(* Logix 5000 AddOnInstructionDefinition export Banner_K50Pro_Compact_Aud_Param_v4; software revision 33.03 *)

TYPE Banner_IOL_Port_v4 :   // UDT that has all of the data items necessary to communicate with a specific Port on a IO-Link Master
STRUCT
   Port_Controlled : INT;   // Each bit represents a port on an IO-Link Master. Set to 1 to tell AOI to control that port.
   Port_Activate : INT;   // Each bit represents a port on an IO-Link Master. When ON that port will process any commands in queue.
   Port_Read : INT;   // Each bit represents a port on an IO-Link Master. Used to determine when device AOI has requested a Read command.
   Port_Write : INT;   // Each bit represents a port on an IO-Link Master. Used to determine when device AOI has requested a Write command.
   Port_RW_Complete : INT;   // Each bit represents a port on an IO-Link Master. Tells device AOI that Read or Write request has been completed.
   Port_Device_Read : INT;
   Data_Transfer : SINT[190];   // Array to transfer data from IO-Master to device AOIs.
END_STRUCT
END_TYPE

TYPE Banner_K50ComAud_Audible_Tone_v4 :   // UDT for K50 Compact Audible with the Custom Audible Tone structure.
STRUCT
   Audible_Type : SINT;   // 0 = Beep, 1 = Sweep, 2 = Tone.
   Sweep_Type : SINT;   // 0 = Up, 1 = Down, 2 = Up Down, 3 = Down Up.
   Frequency1 : SINT;   // 0 = Off, 1 = Low, 2 = Standard, 3 =High.
   Frequency2 : SINT;   // 0 = Off, 1 = Low, 2 = Standard, 3 =High.
END_STRUCT
END_TYPE

TYPE Banner_K50ComAud_Direct_v4 :   // UDT with all of the Direct Parameters for K50 Compact Audible.
STRUCT
   Master_Cycle_Time : INT;
   Min_Cycle_Time : INT;
   M_Sequence_Capability : INT;
   IO_Link_Version_ID : INT;
   Process_Data_Input_Length : INT;
   Process_Data_Output_Length : INT;
   Combined_Vendor_ID : DINT;   // IO-Link Vendor ID
   Vendor_ID1 : INT;
   Vendor_ID2 : INT;
   Combined_Device_ID : DINT;   // IO-Link Device ID
   Device_ID1 : INT;
   Device_ID2 : INT;
   Device_ID3 : INT;
END_STRUCT
END_TYPE

TYPE Banner_K50ComAud_RD_v4 :   // UDT with all of the Read only parameters for K50 Compact Audible.
STRUCT
   Direct : Banner_K50ComAud_Direct_v4;
   Serial_Number : STRING;
END_STRUCT
END_TYPE

TYPE Banner_K50ComAud_SP_v4 :   // UDT for K50 Compact Audible with the State Parameters structure.
STRUCT
   Audible_Feedback : SINT;   // 0 = Off, 3 = On.
   Audible_Volume : SINT;   // 0 = Off, 1 = Low, 2 = Medium, 3 = High.
   Audible_Type : SINT;   // 0 = Pulse, 1 = Wobble, 2 = Strobe, 3 = Whoop, 4 = Stcatto, 5 = Siren, 6 = Continuous 1, 7 = Continuous 2, 9 = Jingle, 10 = Melody 1, 11 = Melody 2, 12 = Melody 3, 13 = Custom.
END_STRUCT
END_TYPE

TYPE Banner_K50ComAud_v4 :   // UDT with all of the parameters for K50 Compact Audible.
STRUCT
   Initial_Global_Read : BOOL;   // Determines if all of the IO-Link data has been read into the PLC yet
   Command : INT;   // Value placed in here will activate a read or write to a specifc IO-Link Index
   Read : Banner_K50ComAud_RD_v4;   // All read data
   Write : Banner_K50ComAud_WD_v4;   // All data that can be written to.
   Reset : BOOL;
END_STRUCT
END_TYPE

TYPE Banner_K50ComAud_WD_v4 :   // UDT that stores the Write Data for a K50 Compact Audible.
STRUCT
   System_Command : INT;   // See IODD file for list of commands that can be activated via the System Command interface
   Parameter_Access_Lock : SINT;   // Write access to all read/write parameters is block when this bit is ON.
   Data_Storage_Lock : SINT;   // Data storage mechanism is inhibited when bit is ON.
   Local_Parameterization_Lock : SINT;   // Parameteriation via local control elementes is inhibited.
   Local_User_Interface_Lock : SINT;   // Operation of the hmi on the device is disabled.
   Operation_Mode : SINT;   // 0 = Multicolor, 1 = Four State Full Logic, 2 = Advanced, 3 = LED Control, 4 = Demo.
   State_Parameters : Banner_K50ComAud_SP_v4[5];   // State Parameters. 1 through 4 will have values.
   Aud_Tone : Banner_K50ComAud_Audible_Tone_v4;   // 0-255. Custom 1 Red.
END_STRUCT
END_TYPE

ADD_ON_INSTRUCTION Banner_K50Pro_Compact_Aud_Param_v4   (* revision 4.0, vendor Banner Engineering *)
// AOI to read and write parameter data to an IO-Link K50 Pro Compact Audible.
VAR_IN_OUT
   K50 : Banner_K50ComAud_v4; {required}
   Port_Data : Banner_IOL_Port_v4; {required}
END_VAR
VAR_INPUT
   Port : DINT; {required}
END_VAR
VAR
   Local_Control : DINT; {access None}
   Global_Read_Command_Value : INT; {access None}
   Global_Write_Command_Value : INT; {access None}
   Command_Being_Processed : BOOL; {access None}
   Index_Write_Control : DINT; {access None}
   Index_Write_Inprocess : INT; {access None}
   Temp_Excess_Gain : DINT[2]; {access None}
   Inprocess_Index : DINT; {access None}
   SP_Index : DINT; {access None}   // State Parameters Index
   SP_Write_Index : DINT; {access None}
   SP_R_Index : DINT; {access None}
   SP_W_Index : DINT; {access None}
END_VAR

ROUTINE Logic   (* ladder *)
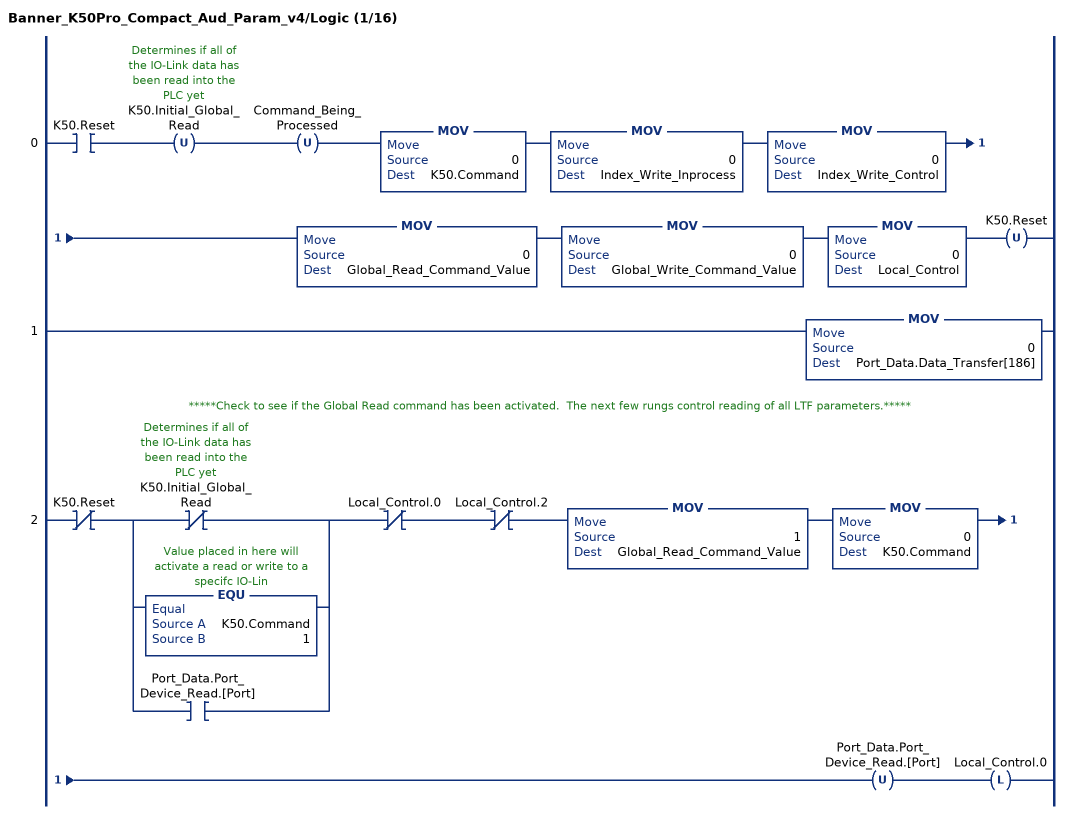
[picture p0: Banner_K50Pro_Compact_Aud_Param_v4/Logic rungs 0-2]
   0: XIC(K50.Reset)OTU(K50.Initial_Global_Read)OTU(Command_Being_Processed)MOV(0,K50.Command)MOV(0,Index_Write_Inprocess)MOV(0,Index_Write_Control)MOV(0,Global_Read_Command_Value)MOV(0,Global_Write_Command_Value)MOV(0,Local_Control)OTU(K50.Reset);
   1: MOV(0,Port_Data.Data_Transfer[186]);
   // *****Check to see if the Global Read command has been activated.  The next few rungs control reading of all LTF parameters.*****
   2: XIO(K50.Reset)[XIO(K50.Initial_Global_Read) ,EQU(K50.Command,1) ,XIC(Port_Data.Port_Device_Read.[Port]) ]XIO(Local_Control.0)XIO(Local_Control.2)MOV(1,Global_Read_Command_Value)MOV(0,K50.Command)OTU(Port_Data.Port_Device_Read.[Port])OTL(Local_Control.0);
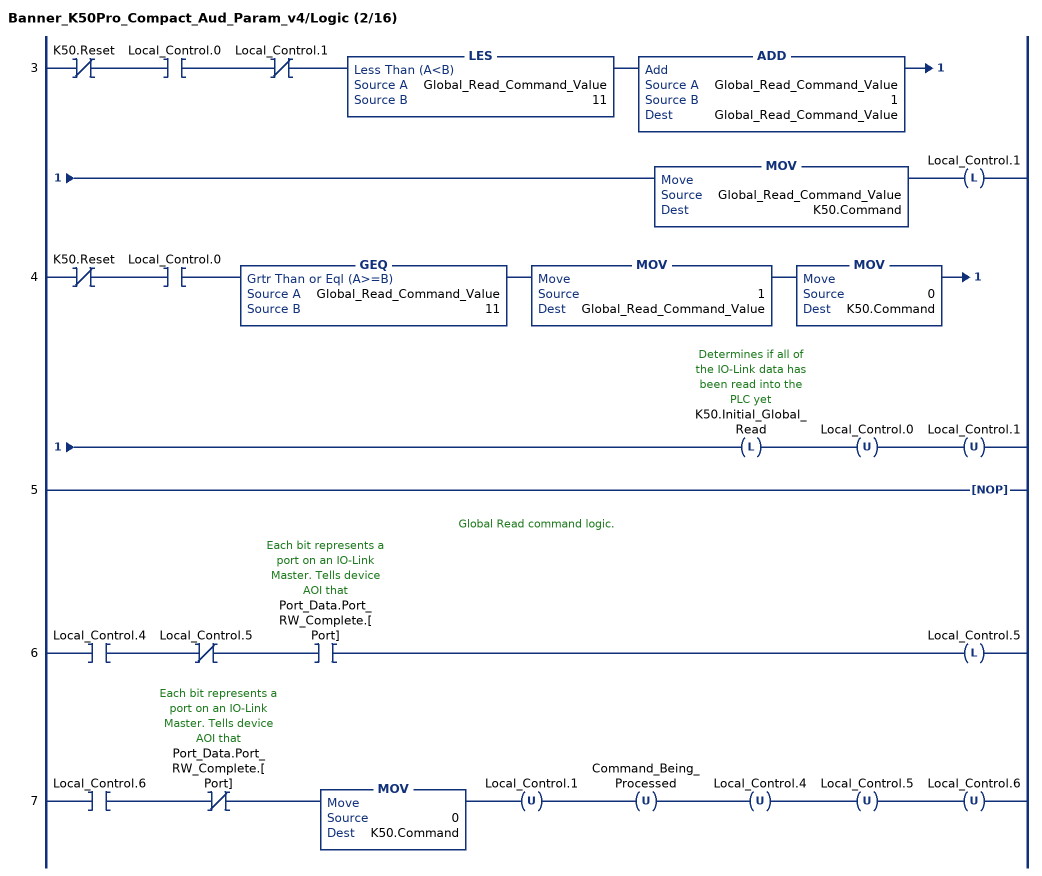
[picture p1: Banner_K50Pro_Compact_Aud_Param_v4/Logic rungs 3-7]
   3: XIO(K50.Reset)XIC(Local_Control.0)XIO(Local_Control.1)LES(Global_Read_Command_Value,11)ADD(Global_Read_Command_Value,1,Global_Read_Command_Value)MOV(Global_Read_Command_Value,K50.Command)OTL(Local_Control.1);
   4: XIO(K50.Reset)XIC(Local_Control.0)GEQ(Global_Read_Command_Value,11)MOV(1,Global_Read_Command_Value)MOV(0,K50.Command)OTL(K50.Initial_Global_Read)OTU(Local_Control.0)OTU(Local_Control.1);
   5: NOP();
   // Global Read command logic.
   6: XIC(Local_Control.4)XIO(Local_Control.5)XIC(Port_Data.Port_RW_Complete.[Port])OTL(Local_Control.5);
   7: XIC(Local_Control.6)XIO(Port_Data.Port_RW_Complete.[Port])MOV(0,K50.Command)OTU(Local_Control.1)OTU(Command_Being_Processed)OTU(Local_Control.4)OTU(Local_Control.5)OTU(Local_Control.6);
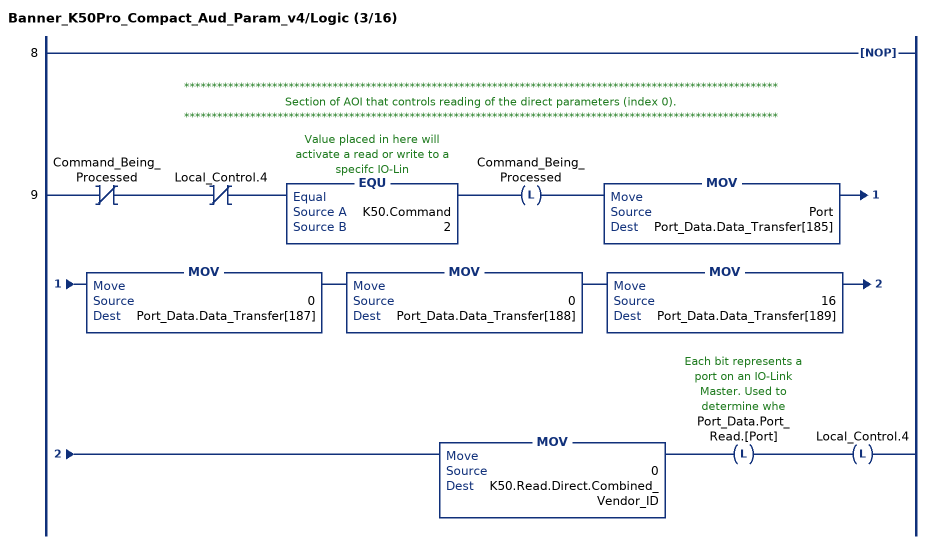
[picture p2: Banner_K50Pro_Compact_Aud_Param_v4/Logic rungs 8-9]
   8: NOP();
   // ************************************************************************************************************
   // Section of AOI that controls reading of the direct parameters (index 0).
   // ************************************************************************************************************
   9: XIO(Command_Being_Processed)XIO(Local_Control.4)EQU(K50.Command,2)OTL(Command_Being_Processed)MOV(Port,Port_Data.Data_Transfer[185])MOV(0,Port_Data.Data_Transfer[187])MOV(0,Port_Data.Data_Transfer[188])MOV(16,Port_Data.Data_Transfer[189])MOV(0,K50.Read.Direct.Combined_Vendor_ID)OTL(Port_Data.Port_Read.[Port])OTL(Local_Control.4);
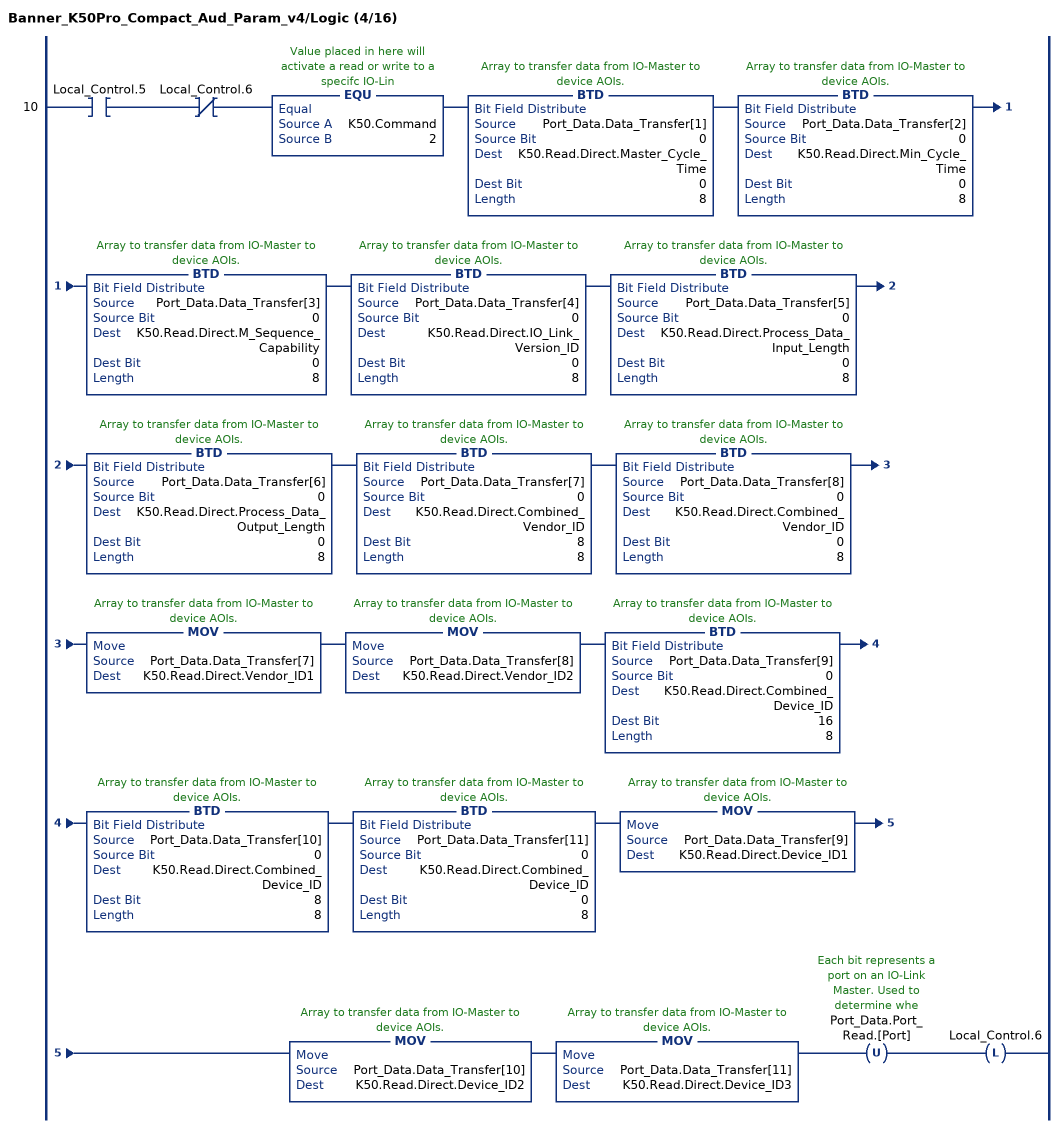
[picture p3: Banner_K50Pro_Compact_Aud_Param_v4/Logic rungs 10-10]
   10: XIC(Local_Control.5)XIO(Local_Control.6)EQU(K50.Command,2)BTD(Port_Data.Data_Transfer[1],0,K50.Read.Direct.Master_Cycle_Time,0,8)BTD(Port_Data.Data_Transfer[2],0,K50.Read.Direct.Min_Cycle_Time,0,8)BTD(Port_Data.Data_Transfer[3],0,K50.Read.Direct.M_Sequence_Capability,0,8)BTD(Port_Data.Data_Transfer[4],0,K50.Read.Direct.IO_Link_Version_ID,0,8)BTD(Port_Data.Data_Transfer[5],0,K50.Read.Direct.Process_Data_Input_Length,0,8)BTD(Port_Data.Data_Transfer[6],0,K50.Read.Direct.Process_Data_Output_Length,0,8)BTD(Port_Data.Data_Transfer[7],0,K50.Read.Direct.Combined_Vendor_ID,8,8)BTD(Port_Data.Data_Transfer[8],0,K50.Read.Direct.Combined_Vendor_ID,0,8)MOV(Port_Data.Data_Transfer[7],K50.Read.Direct.Vendor_ID1)MOV(Port_Data.Data_Transfer[8],K50.Read.Direct.Vendor_ID2)BTD(Port_Data.Data_Transfer[9],0,K50.Read.Direct.Combined_Device_ID,16,8)BTD(Port_Data.Data_Transfer[10],0,K50.Read.Direct.Combined_Device_ID,8,8)BTD(Port_Data.Data_Transfer[11],0,K50.Read.Direct.Combined_Device_ID,0,8)MOV(Port_Data.Data_Transfer[9],K50.Read.Direct.Device_ID1)MOV(Port_Data.Data_Transfer[10],K50.Read.Direct.Device_ID2)MOV(Port_Data.Data_Transfer[11],K50.Read.Direct.Device_ID3)OTU(Port_Data.Port_Read.[Port])OTL(Local_Control.6);
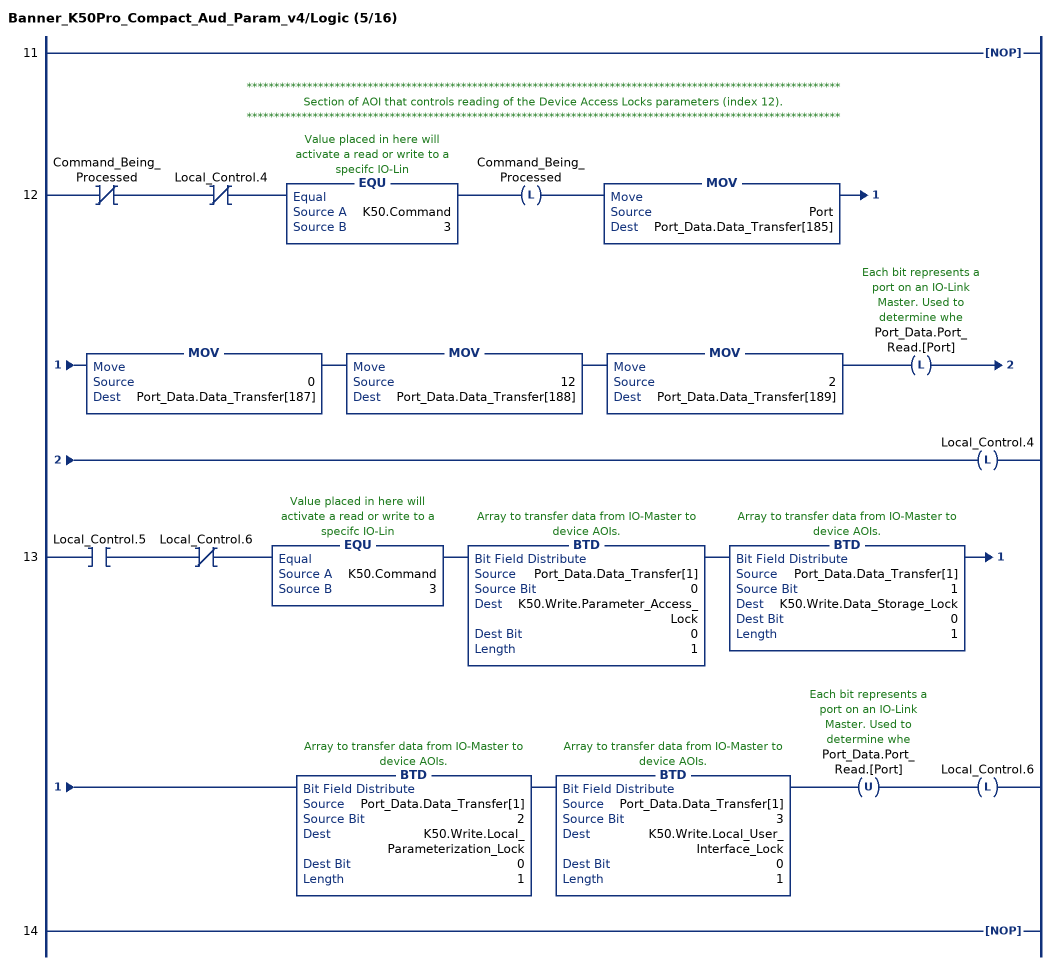
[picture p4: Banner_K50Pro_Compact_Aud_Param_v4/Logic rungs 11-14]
   11: NOP();
   // ************************************************************************************************************
   // Section of AOI that controls reading of the Device Access Locks parameters (index 12).
   // ************************************************************************************************************
   12: XIO(Command_Being_Processed)XIO(Local_Control.4)EQU(K50.Command,3)OTL(Command_Being_Processed)MOV(Port,Port_Data.Data_Transfer[185])MOV(0,Port_Data.Data_Transfer[187])MOV(12,Port_Data.Data_Transfer[188])MOV(2,Port_Data.Data_Transfer[189])OTL(Port_Data.Port_Read.[Port])OTL(Local_Control.4);
   13: XIC(Local_Control.5)XIO(Local_Control.6)EQU(K50.Command,3)BTD(Port_Data.Data_Transfer[1],0,K50.Write.Parameter_Access_Lock,0,1)BTD(Port_Data.Data_Transfer[1],1,K50.Write.Data_Storage_Lock,0,1)BTD(Port_Data.Data_Transfer[1],2,K50.Write.Local_Parameterization_Lock,0,1)BTD(Port_Data.Data_Transfer[1],3,K50.Write.Local_User_Interface_Lock,0,1)OTU(Port_Data.Port_Read.[Port])OTL(Local_Control.6);
   14: NOP();
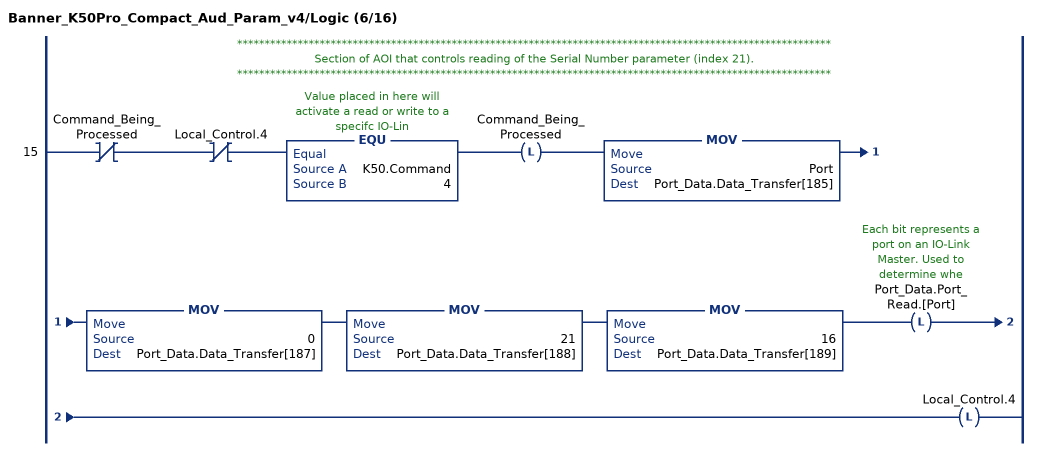
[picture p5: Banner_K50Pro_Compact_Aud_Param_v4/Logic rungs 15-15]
   // ************************************************************************************************************
   // Section of AOI that controls reading of the Serial Number parameter (index 21).
   // ************************************************************************************************************
   15: XIO(Command_Being_Processed)XIO(Local_Control.4)EQU(K50.Command,4)OTL(Command_Being_Processed)MOV(Port,Port_Data.Data_Transfer[185])MOV(0,Port_Data.Data_Transfer[187])MOV(21,Port_Data.Data_Transfer[188])MOV(16,Port_Data.Data_Transfer[189])OTL(Port_Data.Port_Read.[Port])OTL(Local_Control.4);
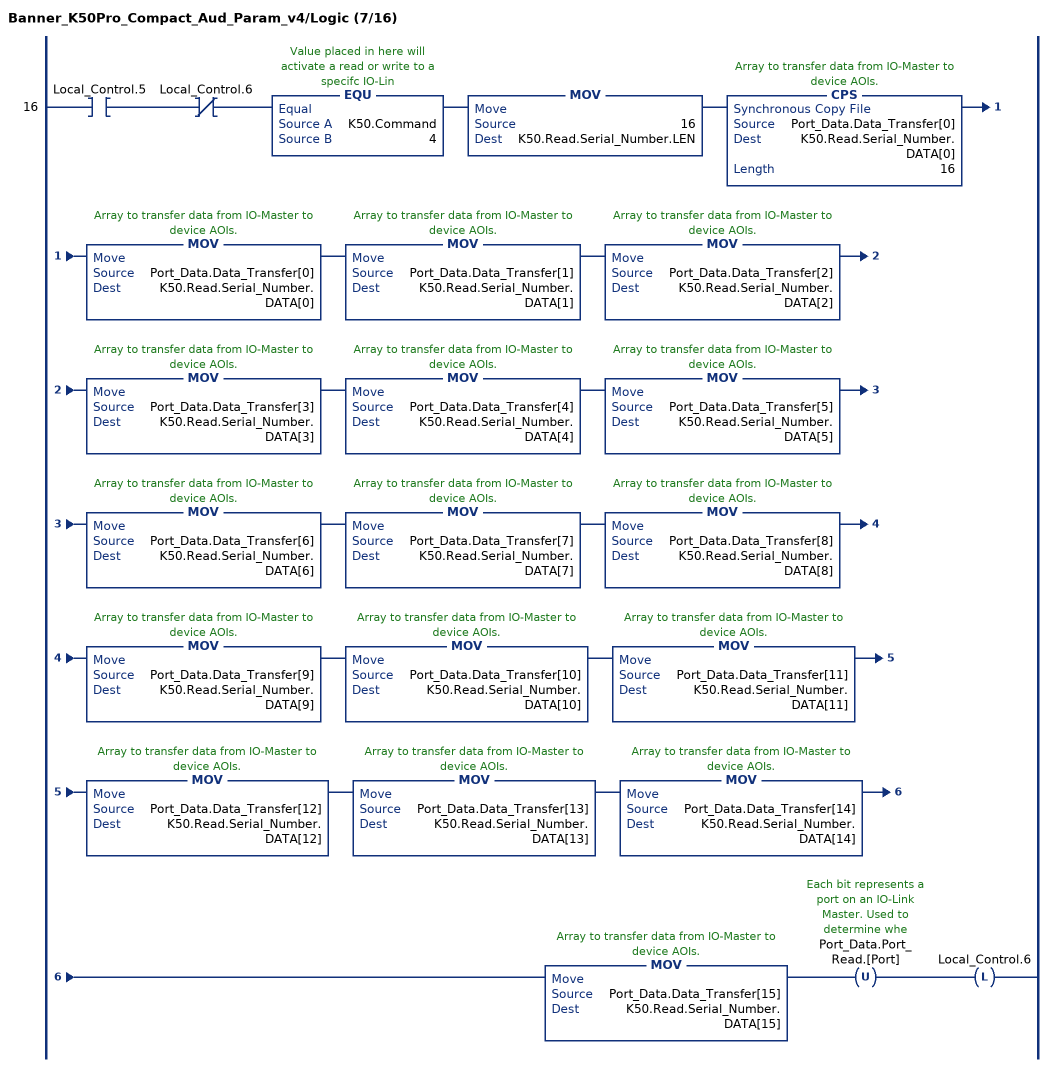
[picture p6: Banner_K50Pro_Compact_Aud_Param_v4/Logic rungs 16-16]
   16: XIC(Local_Control.5)XIO(Local_Control.6)EQU(K50.Command,4)MOV(16,K50.Read.Serial_Number.LEN)CPS(Port_Data.Data_Transfer[0],K50.Read.Serial_Number.DATA[0],16)MOV(Port_Data.Data_Transfer[0],K50.Read.Serial_Number.DATA[0])MOV(Port_Data.Data_Transfer[1],K50.Read.Serial_Number.DATA[1])MOV(Port_Data.Data_Transfer[2],K50.Read.Serial_Number.DATA[2])MOV(Port_Data.Data_Transfer[3],K50.Read.Serial_Number.DATA[3])MOV(Port_Data.Data_Transfer[4],K50.Read.Serial_Number.DATA[4])MOV(Port_Data.Data_Transfer[5],K50.Read.Serial_Number.DATA[5])MOV(Port_Data.Data_Transfer[6],K50.Read.Serial_Number.DATA[6])MOV(Port_Data.Data_Transfer[7],K50.Read.Serial_Number.DATA[7])MOV(Port_Data.Data_Transfer[8],K50.Read.Serial_Number.DATA[8])MOV(Port_Data.Data_Transfer[9],K50.Read.Serial_Number.DATA[9])MOV(Port_Data.Data_Transfer[10],K50.Read.Serial_Number.DATA[10])MOV(Port_Data.Data_Transfer[11],K50.Read.Serial_Number.DATA[11])MOV(Port_Data.Data_Transfer[12],K50.Read.Serial_Number.DATA[12])MOV(Port_Data.Data_Transfer[13],K50.Read.Serial_Number.DATA[13])MOV(Port_Data.Data_Transfer[14],K50.Read.Serial_Number.DATA[14])MOV(Port_Data.Data_Transfer[15],K50.Read.Serial_Number.DATA[15])OTU(Port_Data.Port_Read.[Port])OTL(Local_Control.6);
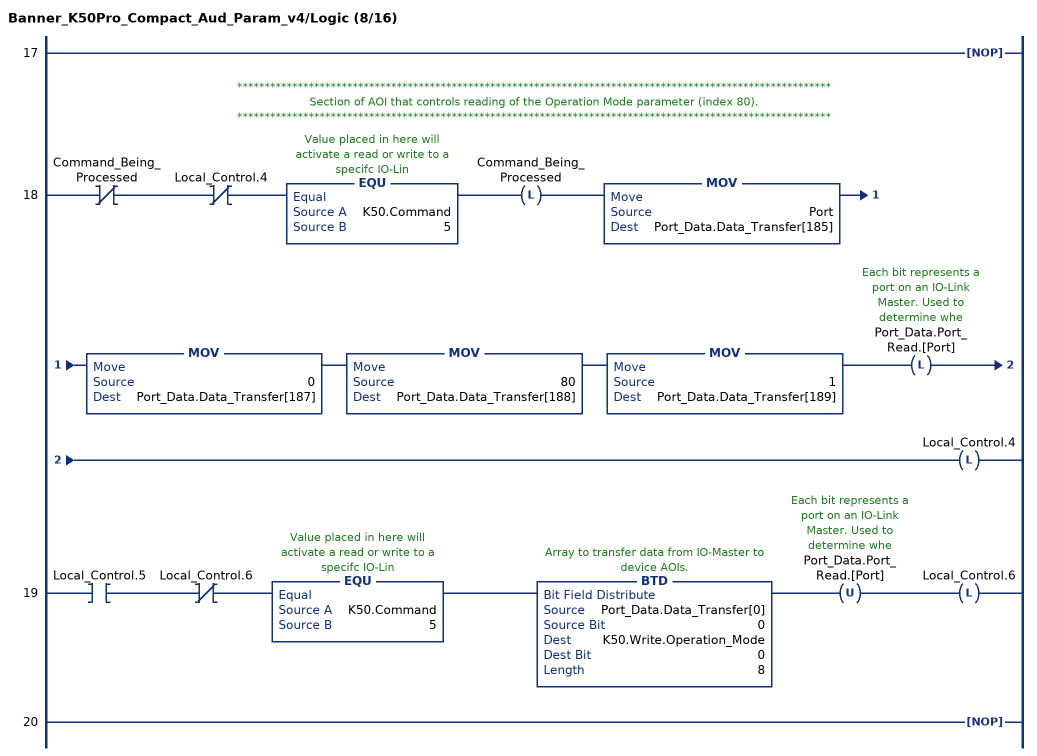
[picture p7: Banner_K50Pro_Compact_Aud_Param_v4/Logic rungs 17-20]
   17: NOP();
   // ************************************************************************************************************
   // Section of AOI that controls reading of the Operation Mode parameter (index 80).
   // ************************************************************************************************************
   18: XIO(Command_Being_Processed)XIO(Local_Control.4)EQU(K50.Command,5)OTL(Command_Being_Processed)MOV(Port,Port_Data.Data_Transfer[185])MOV(0,Port_Data.Data_Transfer[187])MOV(80,Port_Data.Data_Transfer[188])MOV(1,Port_Data.Data_Transfer[189])OTL(Port_Data.Port_Read.[Port])OTL(Local_Control.4);
   19: XIC(Local_Control.5)XIO(Local_Control.6)EQU(K50.Command,5)BTD(Port_Data.Data_Transfer[0],0,K50.Write.Operation_Mode,0,8)OTU(Port_Data.Port_Read.[Port])OTL(Local_Control.6);
   20: NOP();
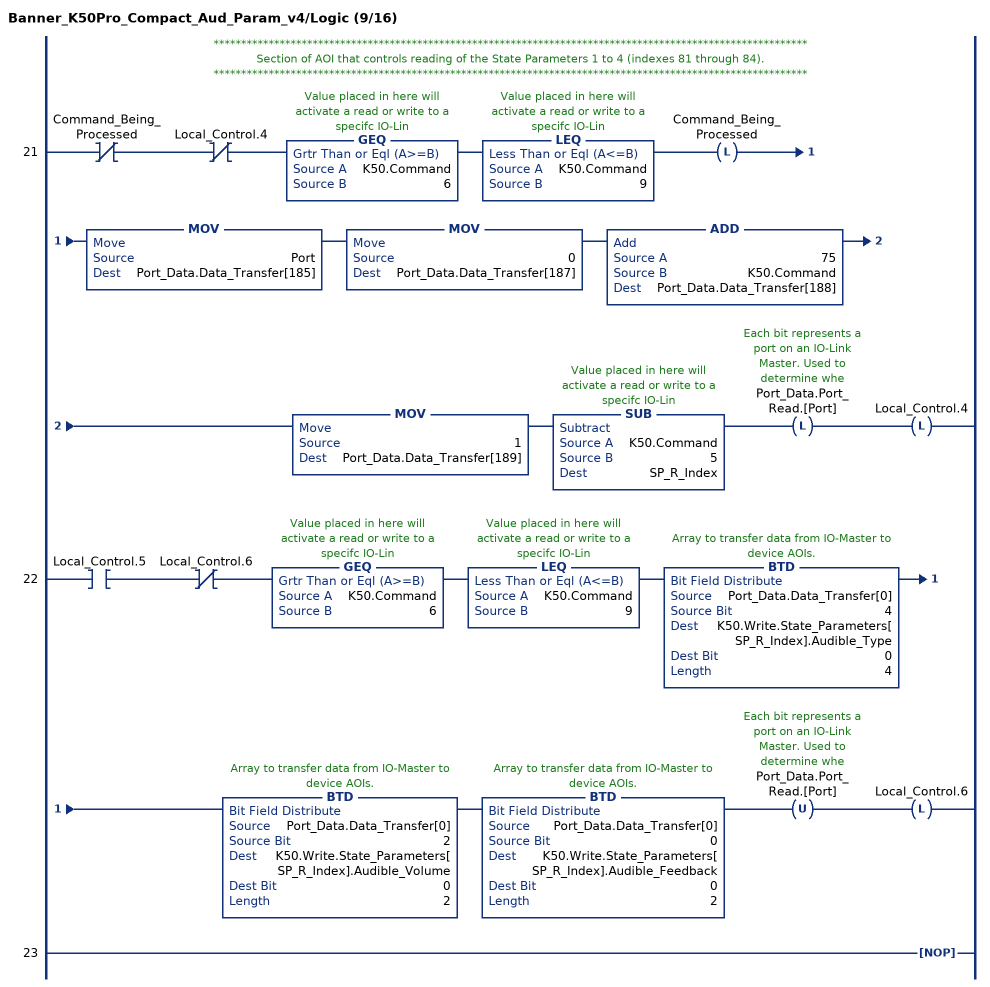
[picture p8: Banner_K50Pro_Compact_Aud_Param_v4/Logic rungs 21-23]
   // ************************************************************************************************************
   // Section of AOI that controls reading of the State Parameters 1 to 4 (indexes 81 through 84).
   // ************************************************************************************************************
   21: XIO(Command_Being_Processed)XIO(Local_Control.4)GEQ(K50.Command,6)LEQ(K50.Command,9)OTL(Command_Being_Processed)MOV(Port,Port_Data.Data_Transfer[185])MOV(0,Port_Data.Data_Transfer[187])ADD(75,K50.Command,Port_Data.Data_Transfer[188])MOV(1,Port_Data.Data_Transfer[189])SUB(K50.Command,5,SP_R_Index)OTL(Port_Data.Port_Read.[Port])OTL(Local_Control.4);
   22: XIC(Local_Control.5)XIO(Local_Control.6)GEQ(K50.Command,6)LEQ(K50.Command,9)BTD(Port_Data.Data_Transfer[0],4,K50.Write.State_Parameters[SP_R_Index].Audible_Type,0,4)BTD(Port_Data.Data_Transfer[0],2,K50.Write.State_Parameters[SP_R_Index].Audible_Volume,0,2)BTD(Port_Data.Data_Transfer[0],0,K50.Write.State_Parameters[SP_R_Index].Audible_Feedback,0,2)OTU(Port_Data.Port_Read.[Port])OTL(Local_Control.6);
   23: NOP();
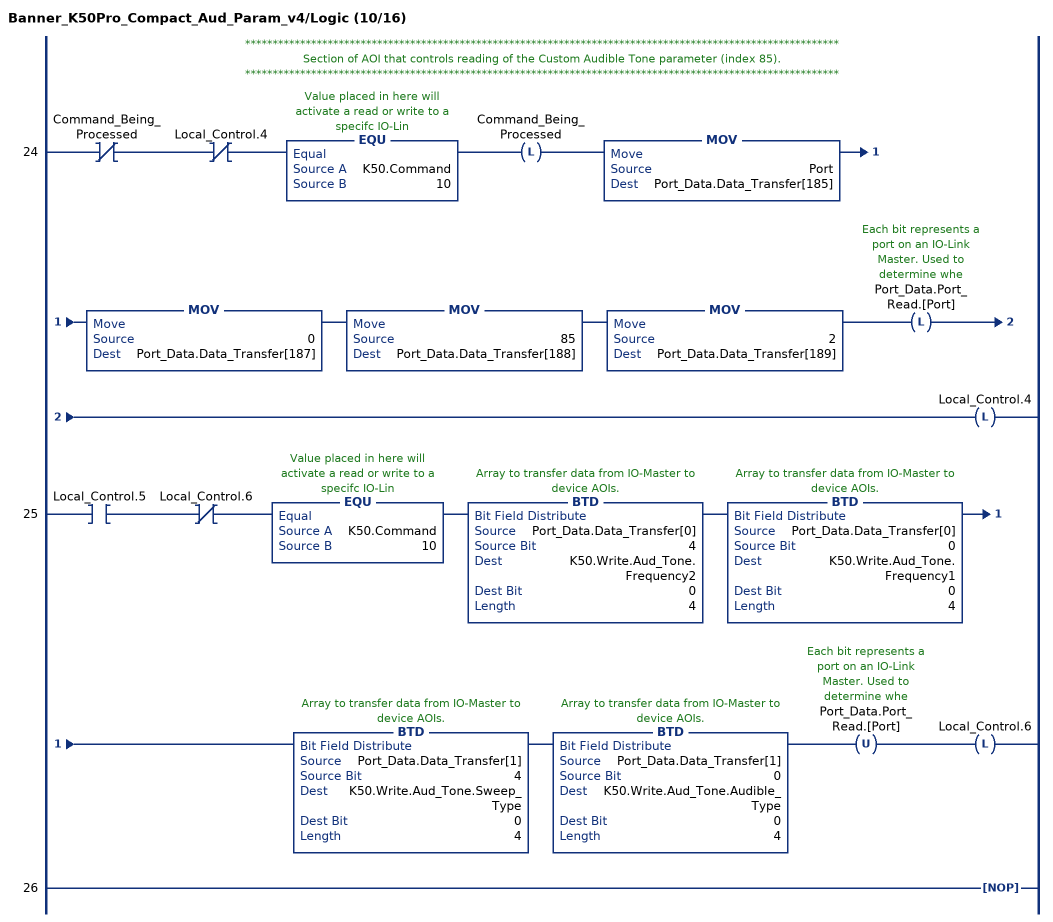
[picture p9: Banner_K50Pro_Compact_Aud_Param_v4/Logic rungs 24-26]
   // ************************************************************************************************************
   // Section of AOI that controls reading of the Custom Audible Tone parameter (index 85).
   // ************************************************************************************************************
   24: XIO(Command_Being_Processed)XIO(Local_Control.4)EQU(K50.Command,10)OTL(Command_Being_Processed)MOV(Port,Port_Data.Data_Transfer[185])MOV(0,Port_Data.Data_Transfer[187])MOV(85,Port_Data.Data_Transfer[188])MOV(2,Port_Data.Data_Transfer[189])OTL(Port_Data.Port_Read.[Port])OTL(Local_Control.4);
   25: XIC(Local_Control.5)XIO(Local_Control.6)EQU(K50.Command,10)BTD(Port_Data.Data_Transfer[0],4,K50.Write.Aud_Tone.Frequency2,0,4)BTD(Port_Data.Data_Transfer[0],0,K50.Write.Aud_Tone.Frequency1,0,4)BTD(Port_Data.Data_Transfer[1],4,K50.Write.Aud_Tone.Sweep_Type,0,4)BTD(Port_Data.Data_Transfer[1],0,K50.Write.Aud_Tone.Audible_Type,0,4)OTU(Port_Data.Port_Read.[Port])OTL(Local_Control.6);
   26: NOP();
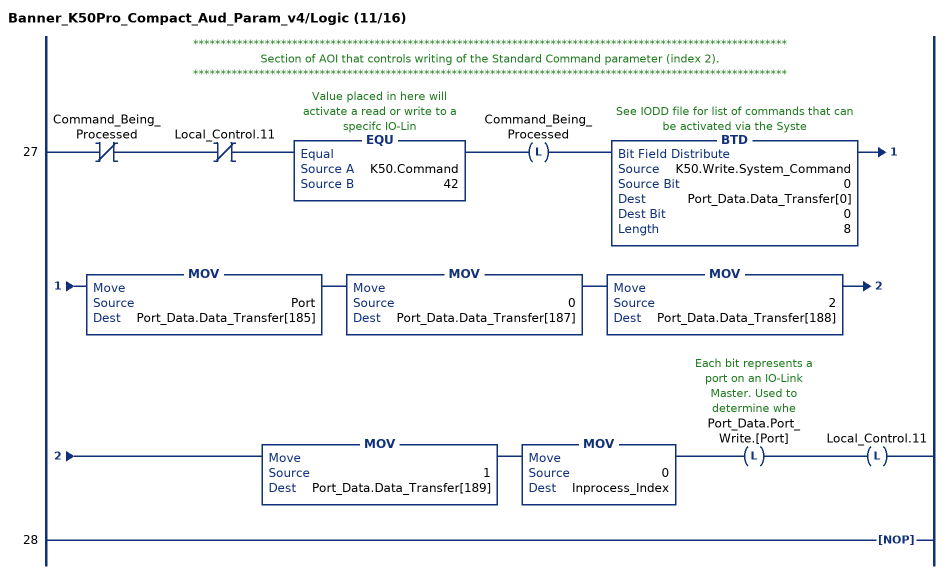
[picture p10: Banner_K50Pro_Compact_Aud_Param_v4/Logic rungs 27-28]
   // ************************************************************************************************************
   // Section of AOI that controls writing of the Standard Command parameter (index 2).
   // ************************************************************************************************************
   27: XIO(Command_Being_Processed)XIO(Local_Control.11)EQU(K50.Command,42)OTL(Command_Being_Processed)BTD(K50.Write.System_Command,0,Port_Data.Data_Transfer[0],0,8)MOV(Port,Port_Data.Data_Transfer[185])MOV(0,Port_Data.Data_Transfer[187])MOV(2,Port_Data.Data_Transfer[188])MOV(1,Port_Data.Data_Transfer[189])MOV(0,Inprocess_Index)OTL(Port_Data.Port_Write.[Port])OTL(Local_Control.11);
   28: NOP();
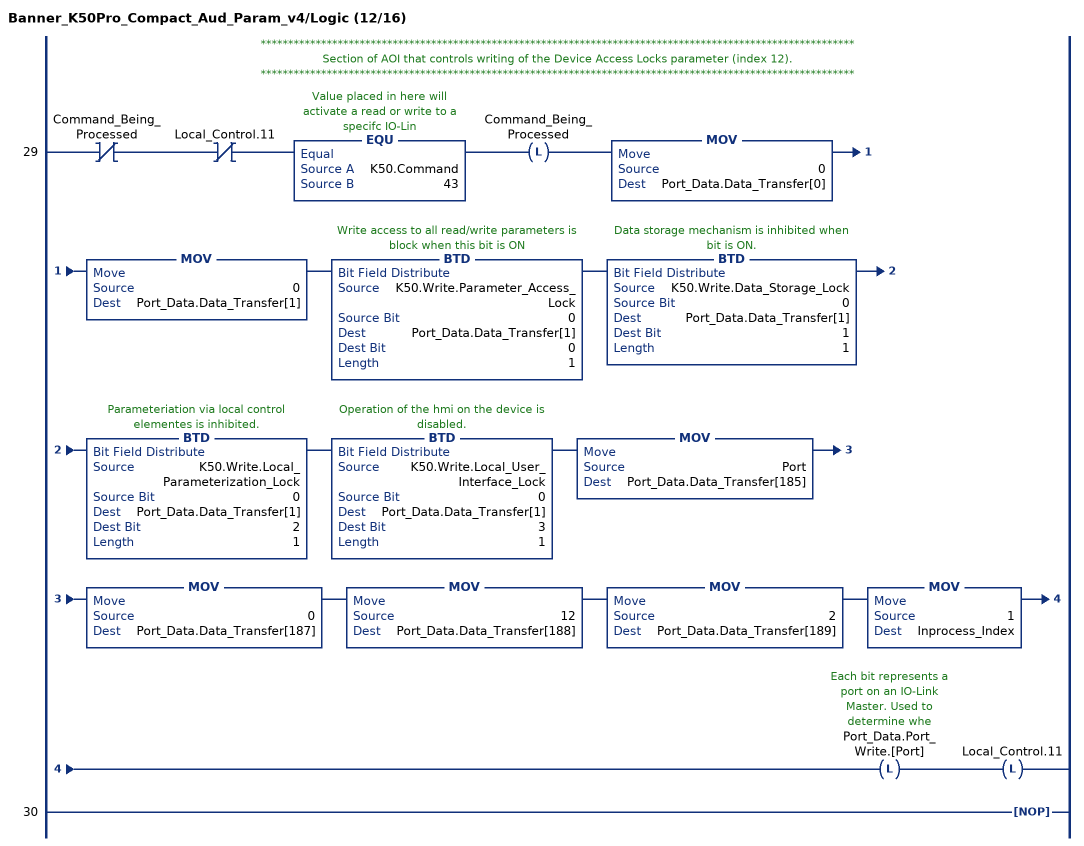
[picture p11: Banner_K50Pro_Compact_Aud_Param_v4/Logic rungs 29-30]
   // ************************************************************************************************************
   // Section of AOI that controls writing of the Device Access Locks parameter (index 12).
   // ************************************************************************************************************
   29: XIO(Command_Being_Processed)XIO(Local_Control.11)EQU(K50.Command,43)OTL(Command_Being_Processed)MOV(0,Port_Data.Data_Transfer[0])MOV(0,Port_Data.Data_Transfer[1])BTD(K50.Write.Parameter_Access_Lock,0,Port_Data.Data_Transfer[1],0,1)BTD(K50.Write.Data_Storage_Lock,0,Port_Data.Data_Transfer[1],1,1)BTD(K50.Write.Local_Parameterization_Lock,0,Port_Data.Data_Transfer[1],2,1)BTD(K50.Write.Local_User_Interface_Lock,0,Port_Data.Data_Transfer[1],3,1)MOV(Port,Port_Data.Data_Transfer[185])MOV(0,Port_Data.Data_Transfer[187])MOV(12,Port_Data.Data_Transfer[188])MOV(2,Port_Data.Data_Transfer[189])MOV(1,Inprocess_Index)OTL(Port_Data.Port_Write.[Port])OTL(Local_Control.11);
   30: NOP();
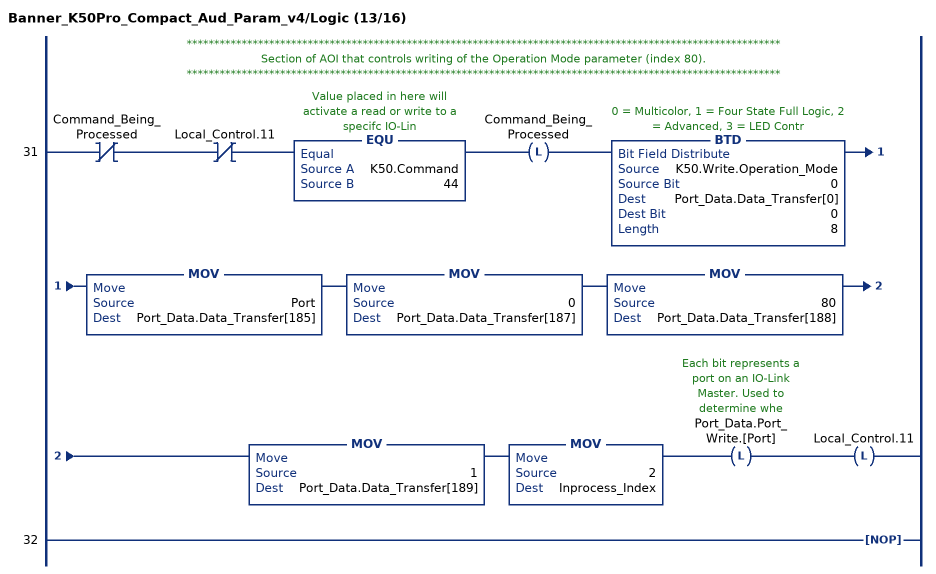
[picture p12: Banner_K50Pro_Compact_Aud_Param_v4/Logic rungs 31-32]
   // ************************************************************************************************************
   // Section of AOI that controls writing of the Operation Mode parameter (index 80).
   // ************************************************************************************************************
   31: XIO(Command_Being_Processed)XIO(Local_Control.11)EQU(K50.Command,44)OTL(Command_Being_Processed)BTD(K50.Write.Operation_Mode,0,Port_Data.Data_Transfer[0],0,8)MOV(Port,Port_Data.Data_Transfer[185])MOV(0,Port_Data.Data_Transfer[187])MOV(80,Port_Data.Data_Transfer[188])MOV(1,Port_Data.Data_Transfer[189])MOV(2,Inprocess_Index)OTL(Port_Data.Port_Write.[Port])OTL(Local_Control.11);
   32: NOP();
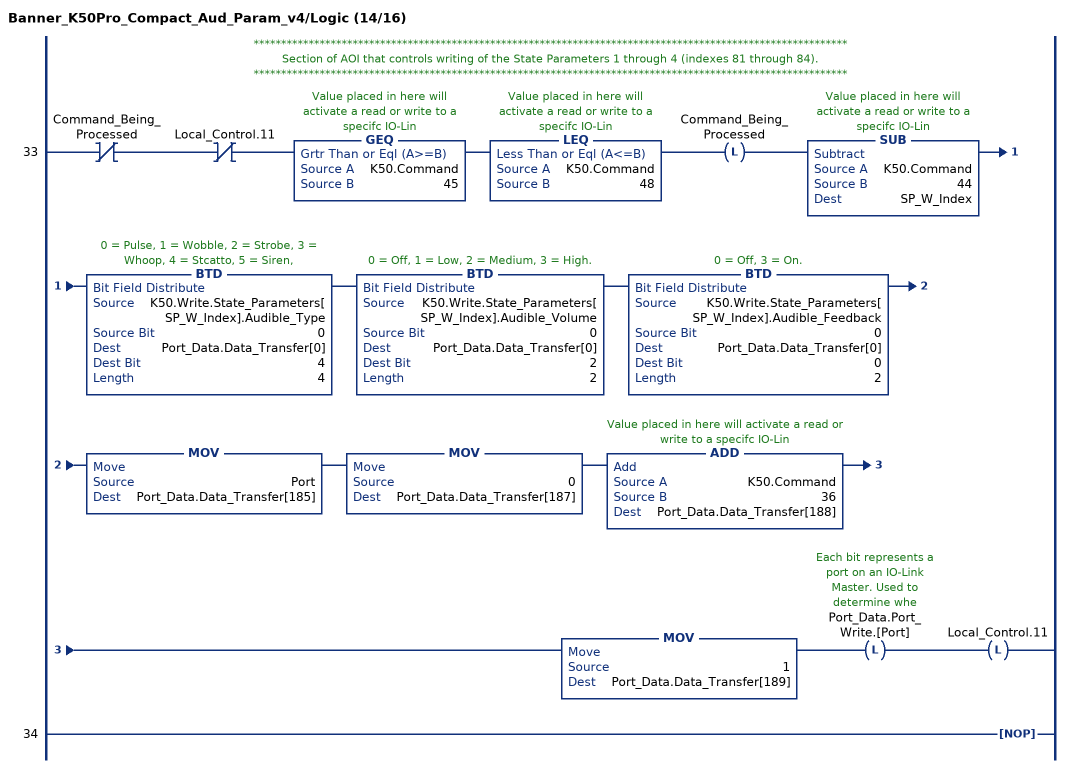
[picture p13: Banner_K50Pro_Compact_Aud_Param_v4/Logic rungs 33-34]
   // ************************************************************************************************************
   // Section of AOI that controls writing of the State Parameters 1 through 4 (indexes 81 through 84).
   // ************************************************************************************************************
   33: XIO(Command_Being_Processed)XIO(Local_Control.11)GEQ(K50.Command,45)LEQ(K50.Command,48)OTL(Command_Being_Processed)SUB(K50.Command,44,SP_W_Index)BTD(K50.Write.State_Parameters[SP_W_Index].Audible_Type,0,Port_Data.Data_Transfer[0],4,4)BTD(K50.Write.State_Parameters[SP_W_Index].Audible_Volume,0,Port_Data.Data_Transfer[0],2,2)BTD(K50.Write.State_Parameters[SP_W_Index].Audible_Feedback,0,Port_Data.Data_Transfer[0],0,2)MOV(Port,Port_Data.Data_Transfer[185])MOV(0,Port_Data.Data_Transfer[187])ADD(K50.Command,36,Port_Data.Data_Transfer[188])MOV(1,Port_Data.Data_Transfer[189])OTL(Port_Data.Port_Write.[Port])OTL(Local_Control.11);
   34: NOP();
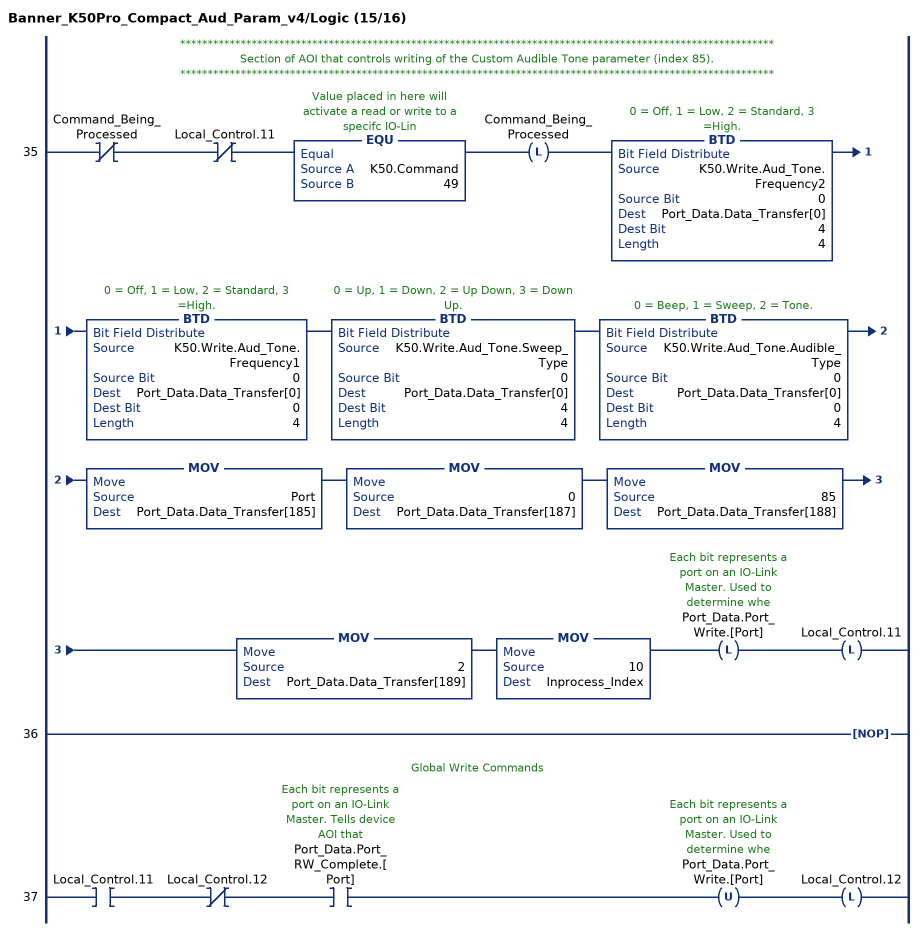
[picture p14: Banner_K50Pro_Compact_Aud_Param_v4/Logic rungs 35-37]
   // ************************************************************************************************************
   // Section of AOI that controls writing of the Custom Audible Tone parameter (index 85).
   // ************************************************************************************************************
   35: XIO(Command_Being_Processed)XIO(Local_Control.11)EQU(K50.Command,49)OTL(Command_Being_Processed)BTD(K50.Write.Aud_Tone.Frequency2,0,Port_Data.Data_Transfer[0],4,4)BTD(K50.Write.Aud_Tone.Frequency1,0,Port_Data.Data_Transfer[0],0,4)BTD(K50.Write.Aud_Tone.Sweep_Type,0,Port_Data.Data_Transfer[0],4,4)BTD(K50.Write.Aud_Tone.Audible_Type,0,Port_Data.Data_Transfer[0],0,4)MOV(Port,Port_Data.Data_Transfer[185])MOV(0,Port_Data.Data_Transfer[187])MOV(85,Port_Data.Data_Transfer[188])MOV(2,Port_Data.Data_Transfer[189])MOV(10,Inprocess_Index)OTL(Port_Data.Port_Write.[Port])OTL(Local_Control.11);
   36: NOP();
   // Global Write Commands
   37: XIC(Local_Control.11)XIO(Local_Control.12)XIC(Port_Data.Port_RW_Complete.[Port])OTU(Port_Data.Port_Write.[Port])OTL(Local_Control.12);
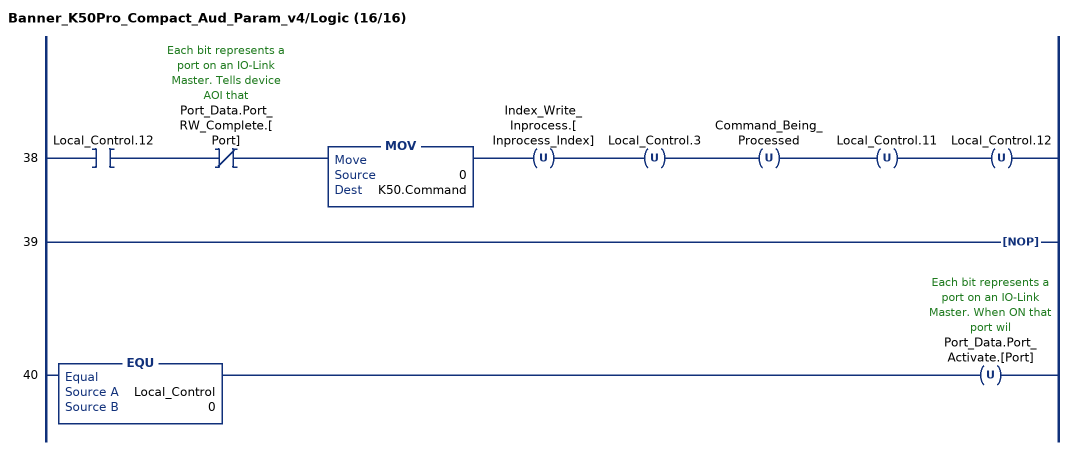
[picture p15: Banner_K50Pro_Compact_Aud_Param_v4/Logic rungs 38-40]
   38: XIC(Local_Control.12)XIO(Port_Data.Port_RW_Complete.[Port])MOV(0,K50.Command)OTU(Index_Write_Inprocess.[Inprocess_Index])OTU(Local_Control.3)OTU(Command_Being_Processed)OTU(Local_Control.11)OTU(Local_Control.12);
   39: NOP();
   40: EQU(Local_Control,0)OTU(Port_Data.Port_Activate.[Port]);
END_ROUTINE
END_ADD_ON_INSTRUCTION
